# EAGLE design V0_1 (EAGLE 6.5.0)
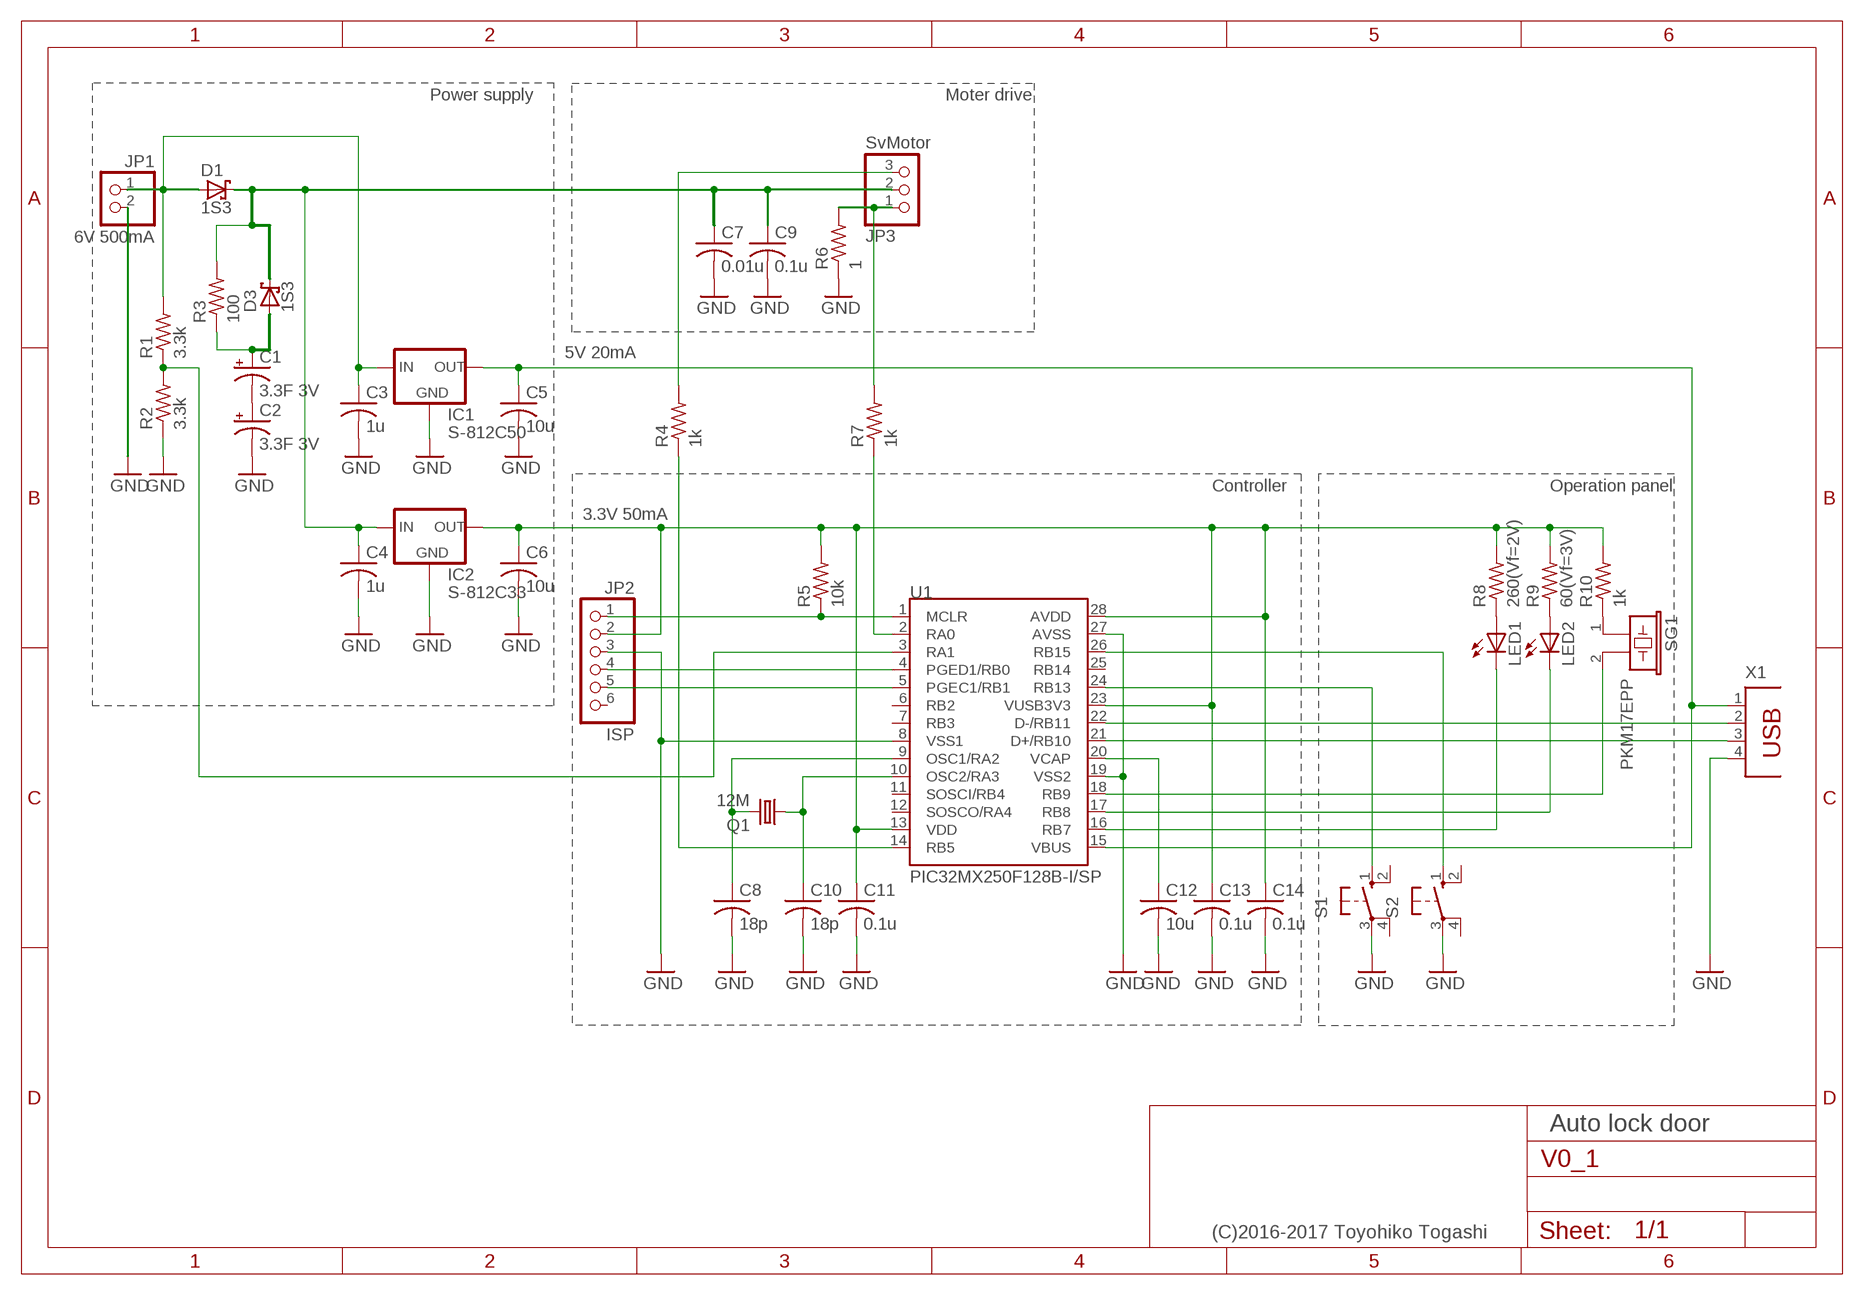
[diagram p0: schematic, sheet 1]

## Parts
C1  3.3F 3V  CPOL-USE10-20  [EB20D]
C2  3.3F 3V  CPOL-USE10-20  [EB20D]
C3  1u  C-US025-024X044  [C025-024X044]
C4  1u  C-US025-024X044  [C025-024X044]
C5  10u  C-US025-024X044  [C025-024X044]
C6  10u  C-US025-024X044  [C025-024X044]
C7  0.01u  C-US050-024X044  [C050-024X044]
C8  18p  C-US025-024X044  [C025-024X044]
C9  0.1u  C-US050-024X044  [C050-024X044]
C10  18p  C-US025-024X044  [C025-024X044]
C11  0.1u  C-US025-024X044  [C025-024X044]
C12  10u  C-US025-024X044  [C025-024X044]
C13  0.1u  C-US025-024X044  [C025-024X044]
C14  0.1u  C-US025-024X044  [C025-024X044]
D1  1S3  SCHOTTKY-DIODEDO35-7  [DO35-7]
D3  1S3  SCHOTTKY-DIODEDO35-7  [DO35-7]
IC1  S-812C50  78LXX  [78LXX]
IC2  S-812C33  78LXX  [78LXX]
JP1  6V 500mA  PINHD-1X2  [1X02]
JP2  ISP  PINHD-1X6  [1X06]
JP3  SvMotor  PINHD-1X3  [1X03]
LED1  LED3MM  [LED3MM]
LED2  LED3MM  [LED3MM]
Q1  12M  CRYSTALHC49S  [HC49/S]
R1  3.3k  R-US_0204/2V  [0204V]
R2  3.3k  R-US_0204/2V  [0204V]
R3  100  R-US_0204/5  [0204/5]
R4  1k  R-US_0204/5  [0204/5]
R5  10k  R-US_0204/2V  [0204V]
R6  1  R-US_0204/5  [0204/5]
R7  1k  R-US_0204/5  [0204/5]
R8  260(Vf=2V)  R-US_0204/5  [0204/5]
R9  60(Vf=3V)  R-US_0204/5  [0204/5]
R10  1k  R-US_0204/5  [0204/5]
S1  10-XX  [B3F-10XX]
S2  10-XX  [B3F-10XX]
SG1  PKM17EPP  [PKM17EPP]
U1  PIC32MX250F128B-I/SP  [DIL28-3]
X1  PN87520  [PN87520]

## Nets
+5V1: C4.1 C7.1 C9.1 D1.C D3.C IC2.IN JP3.2 R3.2
GND: C2.- C3.2 C4.2 C5.2 C6.2 C7.2 C8.2 C9.2 C10.2 C11.2 C12.2 C13.2 C14.2 IC1.GND IC2.GND JP1.2 JP2.3 R2.1 R6.1 S1.3(P) S2.3(P) U1.8(VSS1) U1.19(VSS2) U1.27(AVSS) X1.4
N$1: C8.1 Q1.2 U1.9(OSC1/RA2)
N$2: C10.1 Q1.1 U1.10(OSC2/RA3)
N$3: R4.1 U1.14(RB5)
N$4: JP2.4 U1.4(PGED1/RB0)
N$5: JP2.5 U1.5(PGEC1/RB1)
N$6: C12.1 U1.20(VCAP)
N$7: U1.22(D-/RB11) X1.2
N$8: U1.21(D+/RB10) X1.3
N$9: LED1.A R8.1
N$10: LED1.K(C) U1.16(RB7)
N$11: LED2.A R9.1
N$12: C5.1 IC1.OUT U1.15(VBUS) X1.1
N$13: C1.- C2.+
N$14: R10.1 SG1.1
N$15: LED2.K(C) U1.17(RB8)
N$16: JP3.1 R6.2 R7.2
N$17: S1.1(S) U1.24(RB13)
N$18: S2.1(S) U1.26(RB15)
N$19: JP2.1 R5.1 U1.1(MCLR)
N$20: SG1.2 U1.18(RB9)
N$21: R7.1 U1.2(RA0)
N$22: C6.1 C11.1 C13.1 C14.1 IC2.OUT JP2.2 R5.2 R8.2 R9.2 R10.2 U1.13(VDD) U1.23(VUSB3V3) U1.28(AVDD)
N$23: R1.1 R2.2 U1.3(RA1)
N$24: C3.1 D1.A IC1.IN JP1.1 R1.2
N$25: JP3.3 R4.2
N$27: C1.+ D3.A R3.1
Unconnected: JP2.6 S1.2(S1) S1.4(P1) S2.2(S1) S2.4(P1) U1.6(RB2) U1.7(RB3) U1.11(SOSCI/RB4) U1.12(SOSCO/RA4) U1.25(RB14)

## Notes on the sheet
- Power supply | Moter drive
- 5V 20mA
- Controller | Operation panel
- 3.3V 50mA
- Auto lock door
- (C)2016-2017 Toyohiko Togashi

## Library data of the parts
C1 C2 = rcl:CPOL-US: POLARIZED CAPACITOR, American symbol
C3-C14 = rcl:C-US: CAPACITOR, American symbol
D1 D3 = diode:SCHOTTKY-DIODE: Schottky Diode
IC1 IC2 = v-reg:78LXX: VOLTAGE REGULATOR
JP1 = pinhead:PINHD-1X2: PIN HEADER
JP2 = pinhead:PINHD-1X6: PIN HEADER
JP3 = pinhead:PINHD-1X3: PIN HEADER
LED1 LED2 = led:LED: LED
Q1 = crystal:CRYSTAL: CRYSTAL; OC_FARNELL: 1667008; OC_NEWARK: unknown
R1-R10 = rcl:R-US_: RESISTOR, American symbol
S1 S2 = switch-omron:10-XX: OMRON SWITCH; MPN: B3F-1000; OC_FARNELL: 176432; OC_NEWARK: 36M3542
SG1 = TOG.rpt:PKM17EPP: muRata Piezoelectric Sounder 17mm x 10mm
U1 = TOG.rpt:PIC32MX250F128B
X1 = con-berg:PN87520: BERG USB connector; OC_FARNELL: unknown; OC_NEWARK: unknown

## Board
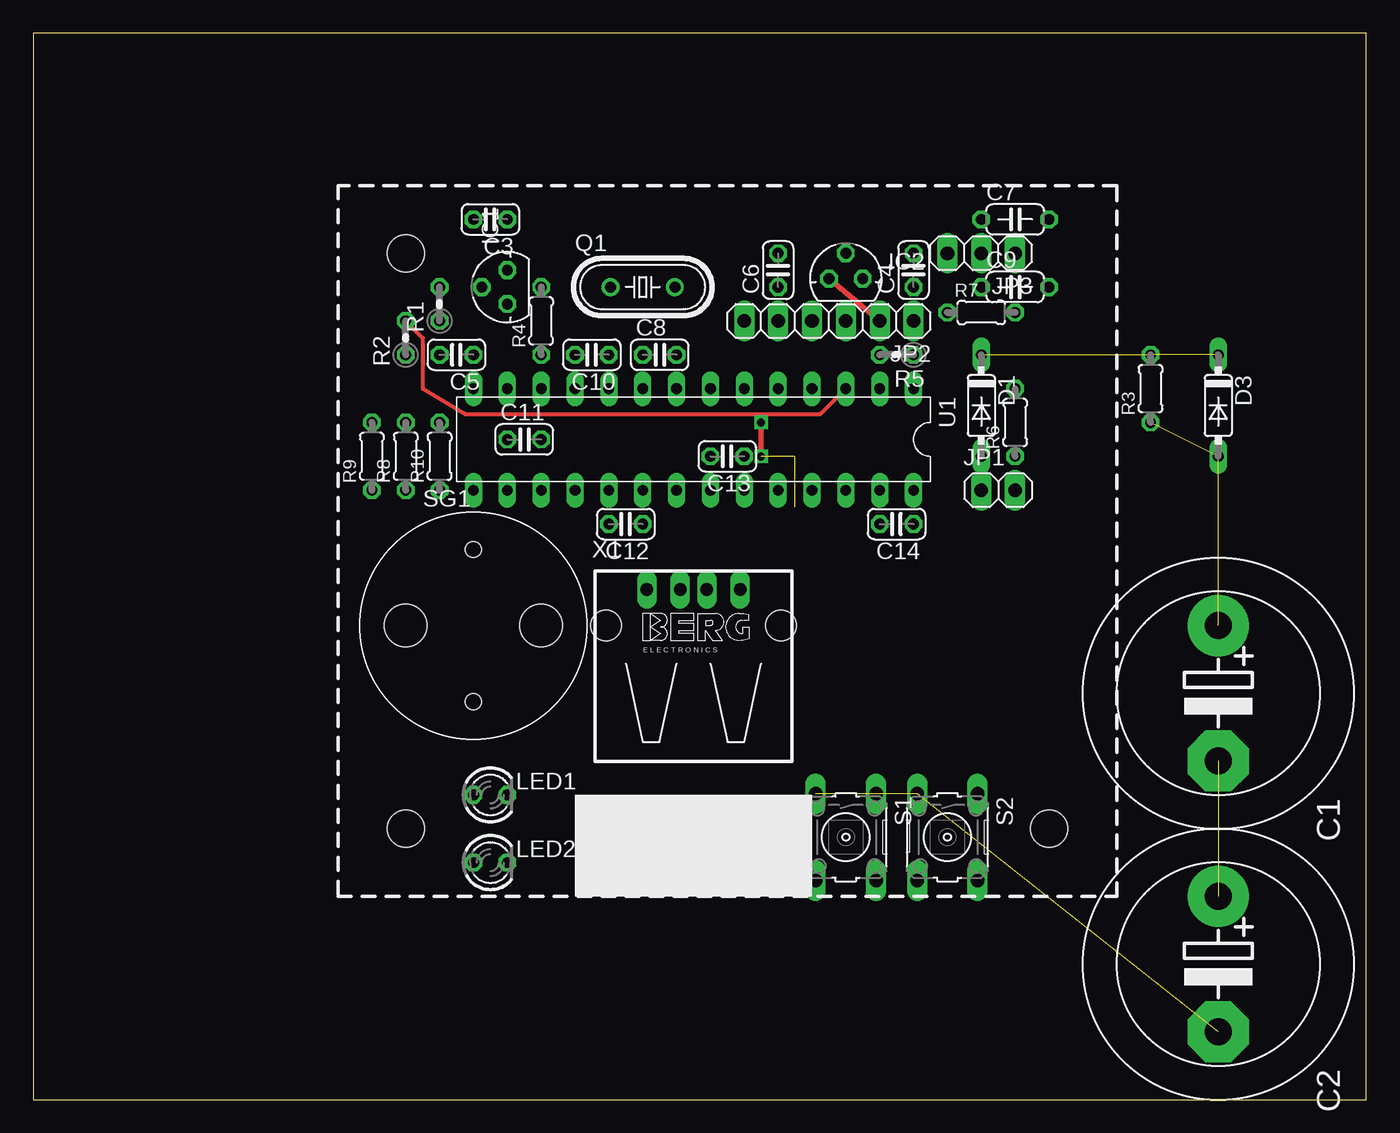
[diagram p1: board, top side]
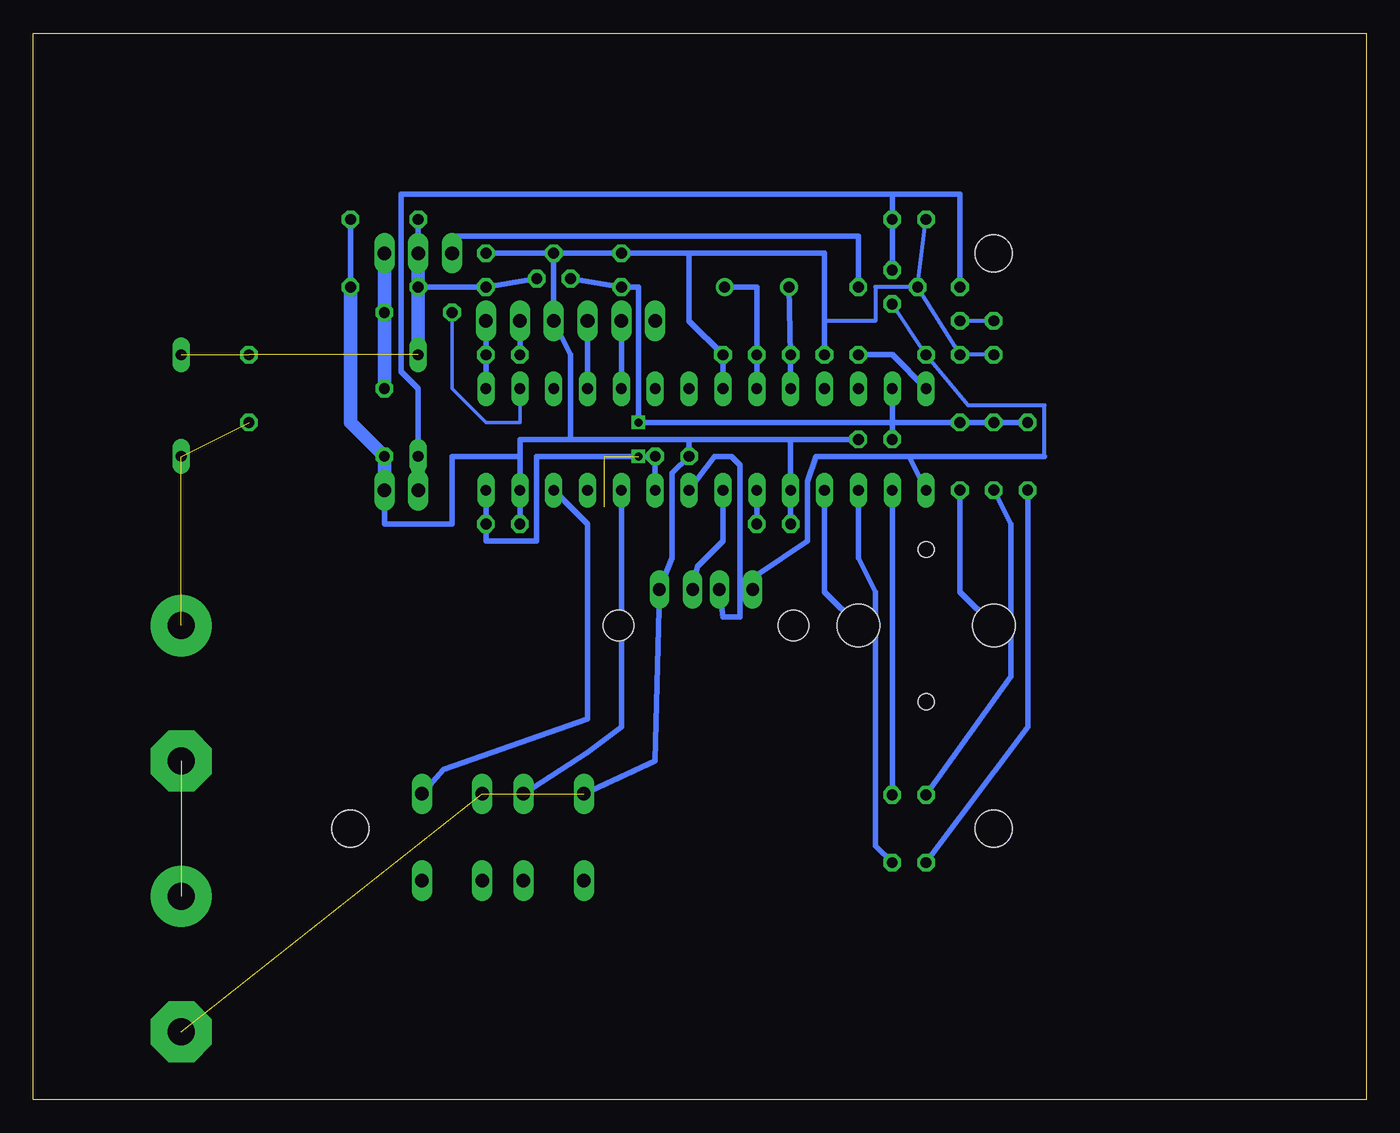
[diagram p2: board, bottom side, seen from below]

Size 100 x 80 mm. Coordinates in mm from the lower left corner, seen from the top.
Outline: 0,0 100,0 100,80 0,80 0,0
Copper layers (1*16): Top 0.035mm / dielectric 1.5mm / Bottom 0.035mm
Design rules "default": minimum track width 10mil, minimum drill 24mil, track to track 8mil, track to pad 8mil, pad to pad 8mil, via to via 8mil, smd to smd 8mil, copper to edge 40mil, drill to drill 8mil, minimum pad ring 10mil, minimum via ring 8mil, stop-mask expansion 4mil, vias tented up to drill 0mil, thermal gap 10mil
Holes 2.8 mm at 76.2,20.32 27.94,20.32 27.94,63.5

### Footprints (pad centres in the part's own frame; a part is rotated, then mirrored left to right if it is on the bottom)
EB20D = drill 2.007 pad 4.597: + -5.08,0 | drill 2.007 pad 4.597 octagon: - 5.08,0
C025-024X044 = drill 0.813 octagon: 1 -1.27,0; 2 1.27,0
C050-024X044 = drill 0.813 octagon: 1 -2.54,0; 2 2.54,0
DO35-7 = drill 0.813 long: A 3.81,0; C -3.81,0
78LXX = drill 0.813 octagon: GND 0,1.905; IN 1.27,0; OUT -1.27,0
1X02 = drill 1.016 long: 1 -1.27,0; 2 1.27,0
1X06 = drill 1.016 long: 1 -6.35,0; 2 -3.81,0; 3 -1.27,0; 4 1.27,0; 5 3.81,0; 6 6.35,0
1X03 = drill 1.016 long: 1 -2.54,0; 2 0,0; 3 2.54,0
LED3MM = drill 0.813 octagon: A -1.27,0; K 1.27,0
HC49/S = drill 0.813: 1 -2.413,0; 2 2.413,0
0204V = drill 0.813 octagon: 1 -1.27,0; 2 1.27,0
0204/5 = drill 0.813 octagon: 1 -2.54,0; 2 2.54,0
B3F-10XX = drill 1.016 long: 1 -3.251,2.261; 2 3.251,2.261; 3 -3.251,-2.261; 4 3.251,-2.261
PKM17EPP = drill 0.8 pad 1.422: 1 -5.08,0; 2 5.08,0 | hole 1.2: 0,5.715; 0,-5.715 | hole 3.2: -5.08,0; 5.08,0
DIL28-3 = drill 0.8 long: 1 -16.51,-3.81; 2 -13.97,-3.81; 3 -11.43,-3.81; 4 -8.89,-3.81; 5 -6.35,-3.81; 6 -3.81,-3.81; 7 -1.27,-3.81; 8 1.27,-3.81; 9 3.81,-3.81; 10 6.35,-3.81; 11 8.89,-3.81; 12 11.43,-3.81; 13 13.97,-3.81; 14 16.51,-3.81; 15 16.51,3.81; 16 13.97,3.81; 17 11.43,3.81; 18 8.89,3.81; 19 6.35,3.81; 20 3.81,3.81; 21 1.27,3.81; 22 -1.27,3.81; 23 -3.81,3.81; 24 -6.35,3.81; 25 -8.89,3.81; 26 -11.43,3.81; 27 -13.97,3.81; 28 -16.51,3.81
PN87520 = drill 0.95 long: 1 -3.5,2.71; 2 -1,2.71; 3 1,2.71; 4 3.5,2.71 | hole 2.3: -6.57,0; 6.57,0

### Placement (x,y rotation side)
C1  88.9,30.48 270 top
C2  88.9,10.16 270 top
C3  34.29,66.04 180 top
C4  66.04,62.23 90 top
C5  31.75,55.88 180 top
C6  55.88,62.23 90 top
C7  73.66,66.04 0 top
C8  46.99,55.88 0 top
C9  73.66,60.96 0 top
C10  41.91,55.88 180 top
C11  36.83,49.53 0 top
C12  44.45,43.18 180 top
C13  52.07,48.26 180 top
C14  64.77,43.18 180 top
D1  71.12,52.07 270 top
D3  88.9,52.07 270 top
IC1  35.56,60.96 90 top
IC2  60.96,61.59 0 top
JP1  72.39,45.72 0 top
JP2  59.69,58.42 180 top
JP3  71.12,63.5 180 top
LED1  34.29,22.86 0 top
LED2  34.29,17.78 0 top
Q1  45.72,60.96 0 top
R1  30.48,59.69 90 top
R2  27.94,57.15 90 top
R3  83.82,53.34 90 top
R4  38.1,58.42 90 top
R5  64.77,55.88 180 top
R6  73.66,50.8 90 top
R7  71.12,59.05 0 top
R8  27.94,48.26 90 top
R9  25.4,48.26 90 top
R10  30.48,48.26 90 top
S1  60.96,19.68 270 top
S2  68.58,19.68 270 top
SG1  33.02,35.56 0 top
U1  49.53,49.53 180 top
X1  49.53,35.56 0 top

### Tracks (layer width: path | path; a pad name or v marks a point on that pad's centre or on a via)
+5V1  (2 unrouted)
  Bottom 0.406: IC2.IN C4.1 C9.1 | C7.1 JP3.2
  Bottom 1.016: JP3.2 C9.1 D1.C
GND  (2 unrouted)
  Bottom 0.305: IC1.GND C3.2 | IC1.GND C5.2 R2.1 | IC1.GND 36.83,60.96 36.83,58.42 40.64,58.42
  Bottom 0.406: U1.8 C8.2 50.8,58.42 50.8,63.5 | 50.8,63.5 40.64,63.5 40.64,58.42 C10.2 | C12.2 U1.19 43.18,49.53 | IC2.GND C6.2 50.8,63.5 | 63.5,48.26 U1.27 C14.2 | 63.5,48.26 63.5,49.53 59.69,49.53 | 59.69,49.53 50.8,49.53 | 43.18,49.53 50.8,49.53 | 50.8,49.53 C13.2 52.07,46.99 52.07,40.64 X1.4 53.34,25.4 S1.3 | C11.2 43.18,49.53 | 59.69,49.53 59.69,55.88 JP2.3 IC2.GND | IC2.GND C4.2 | JP1.2 73.66,43.18 68.58,43.18 68.58,48.26 63.5,48.26 | C7.2 C9.2
  Bottom 1.016: C9.2 76.2,50.8 R6.1 JP1.2
N$1
  Bottom 0.406: U1.9 C8.1 45.72,60.96 Q1.2
N$2
  Bottom 0.406: U1.10 C10.1 Q1.1
N$3
  Bottom 0.406: U1.14 35.56,55.88 R4.1
N$4
  Bottom 0.406: U1.4 JP2.4
N$5
  Bottom 0.406: U1.5 JP2.5
N$6
  Bottom 0.406: U1.20 C12.1
N$7
  Bottom 0.406: X1.2 48.26,36.2 46.99,36.2 46.99,47.62 47.62,48.26 48.9,48.26 U1.22
N$8
  Bottom 0.406: X1.3 50.16,40.01 48.26,41.91 U1.21
N$9
  Bottom 0.406: R8.1 26.67,43.18 26.67,31.75 LED1.A
N$10
  Bottom 0.406: LED1.K U1.16
N$11
  Bottom 0.406: R9.1 25.4,27.94 LED2.A
N$12
  Bottom 0.305: IC1.OUT C5.1 29.84,52.07 24.13,52.07 24.13,48.26
  Bottom 0.406: U1.15 34.29,48.26 | 34.29,48.26 41.27,48.26 41.91,46.35 41.91,41.91 45.72,39.37 X1.1 | 24.13,48.26 34.29,48.26
N$13  (1 unrouted)
N$14
  Bottom 0.406: R10.1 30.48,38.1 SG1.1
N$15
  Bottom 0.406: U1.17 38.1,40.64 36.83,38.1 36.83,19.05 LED2.K
N$16
  Bottom 0.254: R7.2 R6.2
  Bottom 1.016: R6.2 JP3.1
N$17
  Bottom 0.406: S1.1 58.42,26.04 55.88,27.94 U1.24
N$18
  Bottom 0.406: S2.1 69.22,24.77 58.42,28.57 58.42,43.18 U1.26
N$19
  Bottom 0.406: U1.1 R5.1 JP2.1
N$20
  Bottom 0.406: SG1.2 40.64,38.1 U1.18
N$21
  Bottom 0.254: R7.1 68.58,53.34 66.04,50.8 63.5,50.8 U1.2
N$22  (via drill 0.6)  (2 unrouted)
  Top 0.406: JP2.2 IC2.OUT | v54.61,50.8 v54.61,48.26
  Bottom 0.406: IC2.OUT C6.1 54.61,60.96 v54.61,50.8 35.56,50.8 | R9.2 R8.2 R10.2 35.56,50.8 | C11.1 35.56,50.8 | 35.56,50.8 U1.13 | U1.23 C13.1 v54.61,48.26 62.23,48.26 62.23,41.91 66.04,41.91 C14.1 U1.28 | R5.2 JP2.2
N$23
  Top 0.305: U1.3 59.05,51.44 32.38,51.44 29.21,53.34 29.21,57.15 R2.2
  Bottom 0.305: R2.2 R1.1
N$24
  Bottom 0.406: D1.A 71.12,53.34 72.39,54.61 72.39,67.94 35.56,67.94 | 35.56,67.94 30.48,67.94 R1.2 | 35.56,67.94 C3.1 IC1.IN
  Bottom 1.016: D1.A JP1.1
N$25
  Bottom 0.406: R4.2 38.1,64.77 68.58,64.77 JP3.3
N$27  (2 unrouted)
